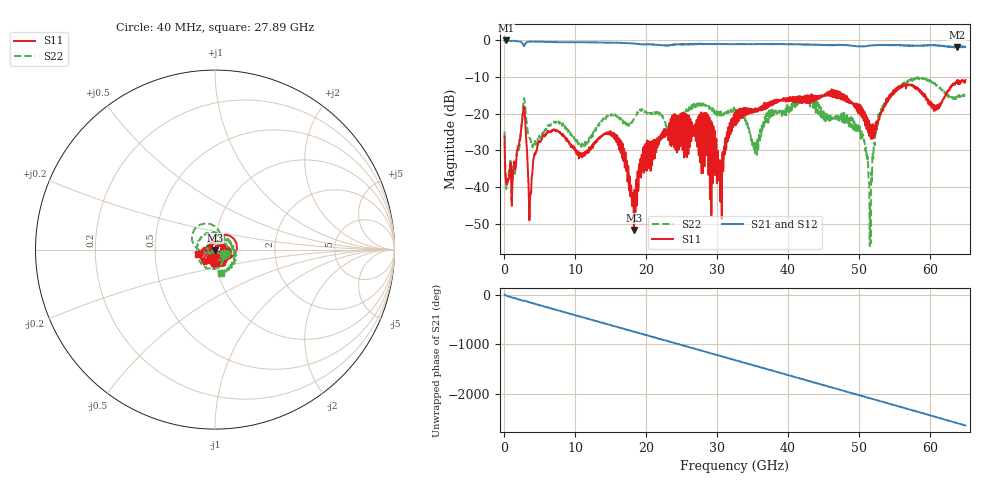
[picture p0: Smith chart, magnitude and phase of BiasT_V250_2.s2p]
! Created Tue Jul 15 19:49:44 2008
# hz S ma R 50
! 2 Port Network Data from blockName block
! freq  magS11  angS11  magS21  angS21  magS12  angS12  magS22  angS22
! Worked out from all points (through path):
!   1601 points, 40 MHz to 65 GHz, reference 50 ohm
!   highest |S21| = -0.09 dB at 243 MHz (marker M1); lowest = -2.0 dB at 63.78 GHz (marker M2)
!   group delay of S21, straight-line fit = 113 ps
!   lowest |S11| = -51.7 dB at 18.27 GHz (marker M3), VSWR 1.01, Z = 50 - j0.256 ohm
!   |S11| at or under -10 dB: start of sweep to end of sweep
!   |S22| runs from -56.2 to -10.0 dB; largest |S21 - S12| = 0.057
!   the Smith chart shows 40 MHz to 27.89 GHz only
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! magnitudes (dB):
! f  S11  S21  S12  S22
! 40 MHz  -26.2  -0.2  -0.2  -24.9
! 243 MHz  -38.8  -0.1  -0.1  -37.8
! 1.299 GHz  -34.5  -0.2  -0.2  -33.4
! 2.801 GHz  -18.2  -1.6  -1.6  -15.8
! 3.653 GHz  -42.2  -0.4  -0.4  -26.9
! 6.089 GHz  -25.2  -0.5  -0.5  -23.7
! 10.88 GHz  -31.0  -0.6  -0.6  -29.1
! 15.43 GHz  -26.7  -0.7  -0.7  -20.4
! 18.27 GHz  -51.7  -0.9  -0.9  -21.5
! 21.72 GHz  -27.0  -1.3  -1.3  -19.6
! 28.42 GHz  -31.0  -1.0  -1.1  -17.8
! 30.45 GHz  -44.1  -1.1  -1.1  -20.5
! 32.52 GHz  -20.3  -1.1  -1.1  -18.8
! 35.48 GHz  -18.8  -1.1  -1.1  -28.0
! 37.59 GHz  -16.8  -1.1  -1.1  -21.1
! 43.36 GHz  -15.7  -1.2  -1.3  -15.9
! 50.02 GHz  -17.9  -1.7  -1.7  -25.4
! 51.52 GHz  -24.0  -1.5  -1.5  -56.2
! 52.62 GHz  -22.4  -1.3  -1.3  -23.4
! 54.2 GHz  -15.6  -1.4  -1.3  -15.8
! 63.78 GHz  -11.3  -2.0  -1.9  -15.4
! 65 GHz  -10.8  -1.8  -2.3  -14.9
